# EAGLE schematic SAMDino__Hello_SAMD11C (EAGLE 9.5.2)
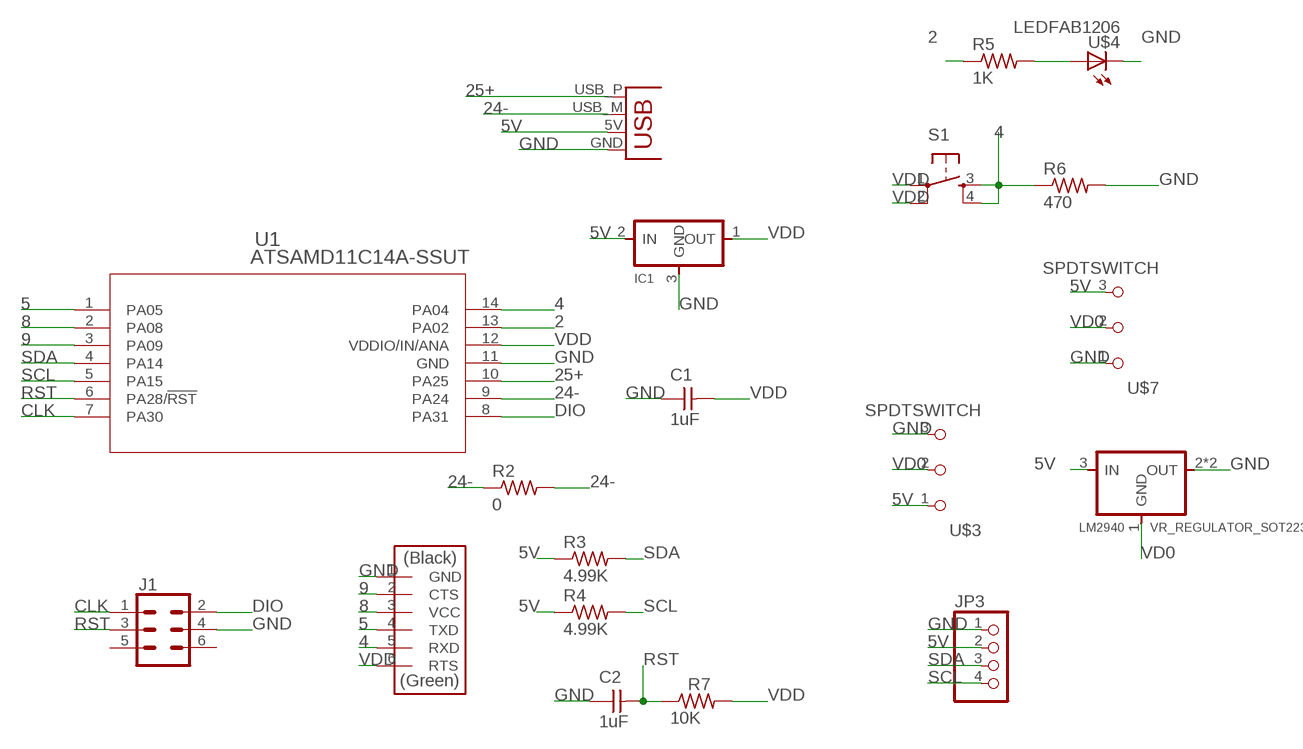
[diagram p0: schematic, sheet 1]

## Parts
C1  1uF  CAP_UNPOLARIZEDFAB  [C1206FAB]
C2  1uF  CAP_UNPOLARIZEDFAB  [C1206FAB]
IC1  VR_REGULATOR-SOT23SOT23  [SOT23]
J1  CONN_03X2SMT  [2X3_SMT_POSTS]
JP3  PINHD-1X04_2.54-SMD-90°  [1X04SMD/90]
LM2940  VR_REGULATOR_SOT223  [SOT223]
R2  0  R1206FAB  [R1206FAB]
R3  4.99K  R1206FAB  [R1206FAB]
R4  4.99K  R1206FAB  [R1206FAB]
R5  1K  R1206FAB  [R1206FAB]
R6  470  RES-US1206FAB  [R1206FAB]
R7  10K  R1206FAB  [R1206FAB]
S1  SW_SWITCH_TACTILE_6MM6MM_SWITCH  [6MM_SWITCH]
U1  ATSAMD11C14A-SSUT  [SOIC14_SL_MCH]
U$3  SPDTSWITCH  [SPDTSWITCH]
U$4  LEDFAB1206  [LED1206FAB]
U$6  CONN_06_FTDI-SMD-HEADER  [1X06SMD]
U$7  SPDTSWITCH  [SPDTSWITCH]
X1  CONN_USBPCB  [USB-A-PCB]

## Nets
2: R5.1 U1.13(PA02)
4: R6.1 S1.3(S) S1.4(S1) U1.14(PA04) U$6.5(RXD)
5: U1.1(PA05) U$6.4(TXD)
5V: IC1.2(IN) JP3.2 LM2940.3(IN) R3.1 R4.1 U$3.1 U$7.3 X1.5V(VBUS)
8: U1.2(PA08) U$6.3(VCC)
9: U1.3(PA09) U$6.2(CTS)
24-: R2.1 R2.2 U1.9(PA24) X1.USB_M(D-)
25+: U1.10(PA25) X1.USB_P(D+)
CLK: J1.1 U1.7(PA30)
DIO: J1.2 U1.8(PA31)
GND: C1.1 C2.1 IC1.3(GND) J1.4 JP3.1 LM2940.2(OUT) LM2940.4(OUT) R6.2 U1.11(GND) U$3.3 U$4.2(C) U$6.1(GND) U$7.1 X1.GND
N$5: R5.2 U$4.1(A)
RST: C2.2 J1.3 R7.1 U1.6(PA28/!RST)
SCL: JP3.4 R4.2 U1.5(PA15)
SDA: JP3.3 R3.2 U1.4(PA14)
VD0: LM2940.1(GND) U$3.2 U$7.2
VDD: C1.2 IC1.1(OUT) R7.2 S1.1(P) S1.2(P1) U1.12(VDDIO/IN/ANA) U$6.6(RTS)
Unconnected: J1.5 J1.6

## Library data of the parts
C1 C2 = fab:CAP_UNPOLARIZED
IC1 = fab:VR_REGULATOR-SOT23
J1 = fab:CONN_03X2: Multi connection point. Often used as Generic Header-pin footprint for 0.1 inch spaced/style header connections You can populate with any combo of single row headers, but if you'd like an exact match, check these: Header - 2x3 (Male, 0.1") (PRT-12807) Header - 2x3 (Female, 0.1") (PRT-13010) 2x3 Pin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; PROD_ID: CONN-11415
JP3 = pinhead-2:PINHD-1X04: PIN HEADER
LM2940 = fab:VR_REGULATOR_SOT223
R2-R5 R7 = fab:R: Resistor (US Symbol)
R6 = fab:RES-US: Resistor (US Symbol)
S1 = fab:SW_SWITCH_TACTILE_6MM: OMRON SWITCH
U1 = samd11c:ATSAMD11C14A-SSUT; BUILT_BY: EMA_Molly; COPYRIGHT: Copyright (C) 2018 Accelerated Designs. All rights reserved; MANUFACTURER_PART_NUMBER: ATSAMD11C14A-SSUT; SOURCELIBRARY: Microchip_2019-08-23_25; VENDOR: Microchip
U$3 U$7 = fab:SPDTSWITCH
U$4 = fab:LED: LED
U$6 = fab:CONN_06_FTDI-SMD-HEADER
X1 = fab:CONN_USB: USB Connectors USB-B-PTH is fully proven SKU : PRT-00139 USB-miniB is fully proven SKU : PRT-00587 USB-A-PCB is untested. USB-A-H is throughly reviewed, but untested. Spark Fun Electronics SKU : PRT-00437 USB-B-SMT is throughly reviewed, but untested. Needs silkscreen touching up. USB-A-S has not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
